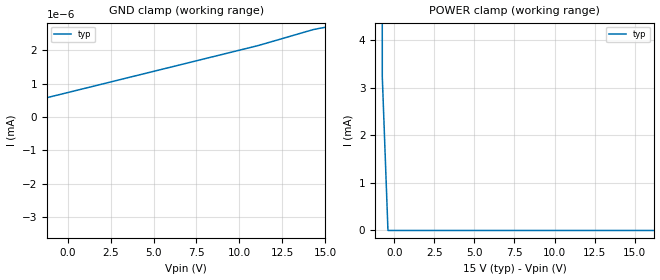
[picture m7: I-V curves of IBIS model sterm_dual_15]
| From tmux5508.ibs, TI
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| sterm_dual_15
[Model]   sterm_dual_15
Model_type   Terminator
|   typ   min   max
C_comp   2.533030e-12   NA   NA
[Voltage Range]   15   NA   NA
[Temperature Range]   27   NA   NA
[Power Clamp Reference]   15   NA   NA
[GND Clamp Reference]   0   NA   NA
[GND Clamp]
|   Voltage   I(typ)   I(min)   I(max)
-20V      -2.839A    NA         NA
-15.4V    -221.5nA   NA         NA
-15.05V   -1.213nA   NA         NA
-14.34V   -1.14nA    NA         NA
-11.16V   -686pA     NA         NA
11.11V    2.144nA    NA         NA
14.29V    2.618nA    NA         NA
15V       2.688nA    NA         NA
[POWER Clamp]
|   Voltage   I(typ)   I(min)   I(max)
-5V       6.669A     NA         NA
-1.111V   236.3mA    NA         NA
-757.6mV  3.236mA    NA         NA
-404mV    187nA      NA         NA
30V       -3.229nA   NA         NA
